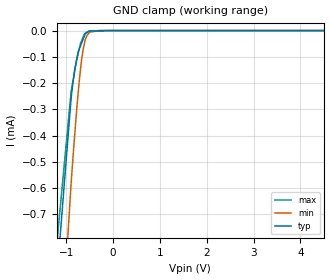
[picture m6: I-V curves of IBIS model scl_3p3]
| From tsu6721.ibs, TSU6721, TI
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|   scl_3p3 Model
[Model]   scl_3p3
Model_type   Input
Vinl = 0.99
Vinh = 2.31
|   typ   min   max
C_comp   1.013e-13   7.984e-14   1.016e-13
[Model spec]
|subparameter
Vinl   0.99   0.9   1.08
Vinh   2.31   2.1   2.52
[Voltage Range]   3.3   3   3.6
|Ambient Temperature   25   85   -40
|Junction Temperature
[Temperature Range]   27   125   -40
[Power Clamp Reference]   3.3   3   3.6
[GND Clamp Reference]   0   0   0
[GND Clamp]
|   Voltage   I(typ)   I(min)   I(max)
-3.3V     -7.436mA   -7.861mA   -7.956mA
-1.332V   -1.237mA   -1.838mA   -1.061mA
-897.6mV  -260.2uA   -586.2uA   -235.6uA
-821.7mV  -151.6uA   -401.5uA   -156uA
-745.8mV  -80.44uA   -237.7uA   -87.33uA
-723mV    -70.2uA    -192.6uA   -70.1uA
-678mV    -49.98uA   -118.9uA   -41.98uA
-636mV    -31.12uA   -67.75uA   -23.63uA
-597mV    -13.6uA    -36.69uA   -10.41uA
-518.4mV  -3.732uA   -10.37uA   -1.786uA
-261mV    -962.2nA   -55.72nA   -87.3nA
6.6V      0A         0A         0A
[POWER Clamp]
|   Voltage   I(typ)   I(min)   I(max)
-3.3V     0A         0A         0A
0V        0A         0A         0A
6.6V      0A         0A         0A
